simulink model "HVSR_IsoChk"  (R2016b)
settings: Solver=VariableStepAuto  StartTime=0.0  StopTime=10.0  RelTol=1e-3
undefined symbols (not defined in the file or in its folder): bin2dec, enmActv, enmBmsMode, enmCctErr, enmSWSta, HVSR_bIsoResShieldCal, HVSR_bSw1EnaByMnl_C, HVSR_bSw2EnaByMnl_C, HVSR_bSw3EnaByMnl_C, HVSR_bSwEnaByMnl_C, HVSR_bVldEnaByMnl_C, HVSR_cntIsoChkCnfDiag_C, HVSR_cntIsoChkCnfLv1Diag_C, HVSR_cntIsoChkDiag_CW, HVSR_cntPwrDown_C, HVSR_cofPosVoltfilter_C, HVSR_cofResGain_C, HVSR_deltInsRes_C, HVSR_InsResCtrlSw_C, HVSR_kSlopeVal_C, HVSR_numBgnTimeCnt_C, HVSR_numCycleTimeCnt_C, HVSR_numIsoCnst_C, HVSR_numSlopeCnfrm_C, HVSR_ResFirstCtrlSw_C, HVSR_resIsoFaultLvl1Thres_C, HVSR_resIsoFaultLvl2Thres_C, HVSR_ResR1_C, HVSR_ResR2_C, HVSR_ResR3_C, HVSR_resRstnUpLim_C, HVSR_rIsoCnfHysDiag_C, HVSR_rIsoCnfHysLv1Diag_C, HVSR_stBMSModeLvl_C, HVSR_tiChkFilteTime_C, HVSR_tiIsoChkCycl_T, HVSR_tiIsoChkDebounce_C, HVSR_tiIsoVldChkDebounce_C, HVSR_tiTaskTime_C, HVSR_tiVoltDiffThres_C, HVSR_uBattVoltRngHi_C, HVSR_uBattVoltRngLo_C, HVSR_uIsoKVoltThres_C, HVSR_uIsoPosVoltFilter_C, HVSR_uIsoVoltThres_C
libraries: simulink x78
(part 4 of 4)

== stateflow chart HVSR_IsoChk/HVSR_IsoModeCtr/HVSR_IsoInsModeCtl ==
  state Stt_init
    entry:
    HVSR_flgIsoChkStart = boolean(0);
    HVSR_stIsoStateObsr=uint8(0);
    HVSR_stIsoCctChkSta = enmCctDiagSta.DEFAULT;
    CctTotalTime = single(0);
  state Stt_CctChk
    entry:
    HVSR_flgIsoChkStart = boolean(0);
    HVSR_stIsoStateObsr=uint8(8);
    CctTotalTime = CctTotalTime+single(0.1);
    during:
    CctTotalTime = CctTotalTime+single(0.1);
    state Stt_CctChkInit
      entry:
      HVSR_stIsoCctChkSta = enmCctDiagSta.INIT;
      HVSR_numA1Val = single(0);
      HVSR_numA2Val = single(0);
      HVSR_numA3Val = single(0);
      HVSR_numA4Val = single(0);
      HVSR_numA5Val = single(0);
      HVSR_flgIsoCctChkOK = boolean(0);
      HVSR_stIsoCctChkErr = enmCctErr.DEFAULT;
      HVSR_bIsoChkSW1Sta = enmSWSta.SWOFF;
      HVSR_bIsoChkSW2Sta = enmSWSta.SWOFF;
      HVSR_bIsoChkSW3Sta = enmSWSta.SWOFF;
      CctCount = single(0);
    state Stt_CctChkA1
      entry:
      CctCount = single(0);
      HVSR_stIsoCctChkSta = enmCctDiagSta.A1CHK;
      HVSR_bIsoChkSW1Sta = enmSWSta.SWOFF;
      HVSR_bIsoChkSW2Sta = enmSWSta.SWOFF;
      HVSR_bIsoChkSW3Sta = enmSWSta.SWOFF;
      HVSR_numA1Val = BSPR_uIsoNegVolt/BSPR_uBattVolt;
      during:
      HVSR_numA1Val = BSPR_uIsoNegVolt/BSPR_uBattVolt;
      CctCount = CctCount + single(0.1);
    state Stt_CctChkA1Err
      entry:
      HVSR_bIsoChkSW1Sta = enmSWSta.SWOFF;
      HVSR_bIsoChkSW2Sta = enmSWSta.SWOFF;
      HVSR_bIsoChkSW3Sta = enmSWSta.SWOFF;
      HVSR_stIsoCctChkErr  = enmCctErr.CCTCLS;
      HVSR_stIsoCctChkSta = enmCctDiagSta.CCTERR;
      %S1或S2或S3常闭粘连
    state Stt_CctChkA2
      entry:
      CctCount = single(0);
      HVSR_stIsoCctChkSta = enmCctDiagSta.A2CHK;
      HVSR_bIsoChkSW1Sta = enmSWSta.SWON;
      HVSR_bIsoChkSW2Sta = enmSWSta.SWOFF;
      HVSR_bIsoChkSW3Sta = enmSWSta.SWOFF;
      HVSR_numA2Val = BSPR_uIsoNegVolt/BSPR_uBattVolt;
      during:
      HVSR_numA2Val = BSPR_uIsoNegVolt/BSPR_uBattVolt;
      CctCount = CctCount + single(0.1);
    state Stt_CctChkA2Err
      entry:
      HVSR_bIsoChkSW1Sta = enmSWSta.SWOFF;
      HVSR_bIsoChkSW2Sta = enmSWSta.SWOFF;
      HVSR_bIsoChkSW3Sta = enmSWSta.SWOFF;
      HVSR_stIsoCctChkErr = enmCctErr.S1ERR;
      HVSR_stIsoCctChkSta = enmCctDiagSta.CCTERR;
      %S1开关回路异常
    state Stt_CctChkA3
      entry:
      CctCount = single(0);
      HVSR_stIsoCctChkSta = enmCctDiagSta.A3CHK;
      HVSR_bIsoChkSW1Sta = enmSWSta.SWOFF;
      HVSR_bIsoChkSW2Sta = enmSWSta.SWON;
      HVSR_bIsoChkSW3Sta = enmSWSta.SWOFF;
      HVSR_numA3Val = BSPR_uIsoNegVolt/BSPR_uBattVolt;
      during:
      HVSR_numA3Val = BSPR_uIsoNegVolt/BSPR_uBattVolt;
      CctCount = CctCount + single(0.1);
    state Stt_CctChkA3Err
      entry:
      HVSR_bIsoChkSW1Sta = enmSWSta.SWOFF;
      HVSR_bIsoChkSW2Sta = enmSWSta.SWOFF;
      HVSR_bIsoChkSW3Sta = enmSWSta.SWOFF;
      HVSR_stIsoCctChkErr = enmCctErr.S2ERR;
      HVSR_stIsoCctChkSta = enmCctDiagSta.CCTERR;
      %S2开关回路异常
    state Stt_CctChkA4
      entry:
      CctCount = single(0);
      HVSR_stIsoCctChkSta = enmCctDiagSta.A4CHK;
      HVSR_bIsoChkSW1Sta = enmSWSta.SWOFF;
      HVSR_bIsoChkSW2Sta = enmSWSta.SWOFF;
      HVSR_bIsoChkSW3Sta = enmSWSta.SWON;
      HVSR_numA4Val = BSPR_uIsoNegVolt/BSPR_uBattVolt;
      during:
      HVSR_numA4Val = BSPR_uIsoNegVolt/BSPR_uBattVolt;
      CctCount = CctCount + single(0.1);
    state Stt_CctChkA4Err
      entry:
      CctCount = single(0);
      HVSR_stIsoCctChkSta = enmCctDiagSta.A5CHK;
      HVSR_bIsoChkSW1Sta = enmSWSta.SWON;
      HVSR_bIsoChkSW2Sta = enmSWSta.SWOFF;
      HVSR_bIsoChkSW3Sta = enmSWSta.SWON;
      HVSR_numA5Val = BSPR_uIsoNegVolt/BSPR_uBattVolt;
      during:
      HVSR_numA5Val = BSPR_uIsoNegVolt/BSPR_uBattVolt;
      CctCount = CctCount + single(0.1);
    state Stt_CctChkA5
      entry:
      HVSR_stIsoCctChkSta = enmCctDiagSta.A5CHK;
      HVSR_bIsoChkSW1Sta = enmSWSta.SWOFF;
      HVSR_bIsoChkSW2Sta = enmSWSta.SWOFF;
      HVSR_bIsoChkSW3Sta = enmSWSta.SWOFF;
      HVSR_flgIsoCctChkOK = boolean(1);
      HVSR_stIsoCctChkErr = enmCctErr.DEFAULT;
      %HVSR_stIsoCctChkErr = enmCctErr.S3ERR;
      HVSR_stIsoCctChkSta = enmCctDiagSta.CCTERR;
      %S3合不上或者Rp和Rn都非常大
    state Stt_CctChkA4OK
      entry:
      CctCount = single(0);
      HVSR_stIsoCctChkSta = enmCctDiagSta.A4CHK;
      HVSR_bIsoChkSW1Sta = enmSWSta.SWOFF;
      HVSR_bIsoChkSW2Sta = enmSWSta.SWOFF;
      HVSR_bIsoChkSW3Sta = enmSWSta.SWOFF;
    state Stt_CctChkA4OKRn
      entry:
      CctCount = single(0);
      HVSR_stIsoCctChkSta = enmCctDiagSta.CCTOK;
      HVSR_bIsoChkSW1Sta = enmSWSta.SWOFF;
      HVSR_bIsoChkSW2Sta = enmSWSta.SWOFF;
      HVSR_bIsoChkSW3Sta = enmSWSta.SWOFF;
      HVSR_flgIsoCctChkOK = boolean(1);
    state Stt_CctChkA4OKRp
      entry:
      CctCount = single(0);
      HVSR_stIsoCctChkSta = enmCctDiagSta.CCTOK;
      HVSR_bIsoChkSW1Sta = enmSWSta.SWOFF;
      HVSR_bIsoChkSW2Sta = enmSWSta.SWOFF;
      HVSR_bIsoChkSW3Sta = enmSWSta.SWOFF;
      HVSR_flgIsoCctChkOK = boolean(1);
    (default) -> Stt_CctChkInit
    Stt_CctChkInit -> Stt_CctChkA1
    Stt_CctChkA1 -> Stt_CctChkA1Err : [CctCount >HVSR_tiIsoCctChkWait_T]
    Stt_CctChkA1 -> Stt_CctChkA2 : [HVSR_numA1Val >=HVSR_numSwAllOpenMin_C &&...  HVSR_numA1Val <=HVSR_numSwAllOpenMax_C]
    Stt_CctChkA2 -> Stt_CctChkA2Err : [CctCount >HVSR_tiIsoCctChkWait_T]
    Stt_CctChkA2 -> Stt_CctChkA3 : [(HVSR_numA2Val >=HVSR_numSw1ClsdMin_C &&...  HVSR_numA2Val <=HVSR_numSw1ClsdMax_C)&&...  ((HVSR_numA2Val-HVSR_numA1Val) >= HVSR_numA1A2DiffMin_C &&... (HVSR_numA2Val-HVSR_numA1Val) <= HVSR_numA1A2DiffMax_C)]
    Stt_CctChkA3 -> Stt_CctChkA3Err : [CctCount >HVSR_tiIsoCctChkWait_T]
    Stt_CctChkA3 -> Stt_CctChkA4 : [(HVSR_numA3Val >=HVSR_numSw2ClsdMin_C &&...  HVSR_numA3Val <=HVSR_numSw2ClsdMax_C)&&... ((HVSR_numA1Val-HVSR_numA3Val) >= HVSR_numA1A3DiffMin_C &&... (HVSR_numA1Val-HVSR_numA3Val) <= HVSR_numA1A3DiffMax_C)]
    Stt_CctChkA4 -> Stt_CctChkA4Err : [CctCount >HVSR_tiIsoCctChkWait_T]
    Stt_CctChkA4 -> Stt_CctChkA4OK : [abs(HVSR_numA4Val-HVSR_numA1Val) >= HVSR_numA1A4Diff_C]
    Stt_CctChkA4Err -> Stt_CctChkA5 : [HVSR_numA5Val >=HVSR_numSw13ClsdMin_C &&...  HVSR_numA5Val <=HVSR_numSw13ClsdMax_C]
    Stt_CctChkA4OK -> (junction 191)
    (junction 191) -> Stt_CctChkA4OKRp
    Stt_CctChkA4OK -> Stt_CctChkA4OKRn : [(HVSR_numA4Val-HVSR_numA1Val) >= HVSR_numA1A4Diff_C]
  state Stt_fastchk
    entry:
    HVSR_flgIsoChkStart = boolean(0);
    HVSR_stIsoStateObsr=uint8(7);
  state Stt_standby
    entry:
    init_enable = enmActv.ACTIVE;
    begin_enable=enmActv.INACTIVE;
    control_enable=enmActv.INACTIVE;
    HVSR_flgIsoChkFault = boolean(0);
    HVSR_flgIsoChkStart = boolean(0);
    HVSR_stIsoStateObsr=uint8(1);
  state Stt_begin
    entry:
    init_enable = enmActv.INACTIVE;
    begin_enable=enmActv.ACTIVE;
    control_enable=enmActv.INACTIVE;
    HVSR_flgIsoChkStart = boolean(1);
    HVSR_flgInsResUpd = boolean(0);
    HVSR_stIsoStateObsr=uint8(2);
    counter = uint16(1);
    during:
    counter = counter + uint16(1);
  state Stt_work
    entry:
    init_enable = enmActv.INACTIVE;
    begin_enable=enmActv.INACTIVE;
    control_enable=enmActv.ACTIVE;
    HVSR_stIsoStateObsr=uint8(3);
  state Stt_fault
    entry:
    HVSR_flgIsoChkFault = boolean(1);
    HVSR_stIsoStateObsr=uint8(5);
  state 300 [group]
  state Stt_cycle
    entry:
    HVSR_flgInsResUpd = boolean(1);
    HVSR_flgIsoChkFault = boolean(0);
    HVSR_stIsoStateObsr=uint8(4);
    count = uint16(0);
    during:
    count =count + uint16(1);
  state Stt_end
    entry:
    init_enable = enmActv.ACTIVE;
    begin_enable=enmActv.INACTIVE;
    control_enable=enmActv.INACTIVE;
    HVSR_flgIsoChkStart = boolean(0);
    HVSR_stIsoStateObsr=uint8(6);
  (default) -> Stt_init
  Stt_init -> Stt_CctChk : [(BMCR_stBmsModeCtrl >= uint8(2))&&(BMCR_stBmsModeCtrl<=HVSR_ModLvl_C)]
  Stt_CctChk -> Stt_fastchk : [boolean(1) == HVSR_flgIsoCctChkOK||... CctTotalTime >= HVSR_tiIsoCctChkTotMax_T||... HVSR_bIsoCctChkEna_C]
  Stt_fastchk -> Stt_standby
  (junction 115) -> Stt_standby
  (junction 112) -> (junction 115)
  Stt_standby -> Stt_begin : [IsoResCalShieldCmd==boolean(0)]
  Stt_begin -> (junction 112) : [IsoResCalShieldCmd==1]
  (junction 109) -> (junction 112)
  (junction 86) -> Stt_begin
  (junction 50) -> Stt_begin
  Stt_fault -> (junction 86) : [BMCR_stBmsModeCtrl<=HVSR_ModLvl_C]
  (junction 48) -> (junction 50)
  Stt_begin -> (junction 47) : [(counter>HVSR_BgTi_C)&&(HVSR_flgFrstRsVlotVld==1)]
  (junction 47) -> Stt_work : {HVSR_cntPwrDown = uint16(0)}
  (junction 43) -> Stt_work : {HVSR_cntPwrDown = HVSR_cntPwrDown + 1}
  (junction 39) -> (junction 43)
  Stt_work -> Stt_fault : [(flgResVald == 0)&&(HVSR_cntPwrDown > HVSR_cntPwrDown_C)]
  Stt_work -> (junction 39) : [(flgResVald == 0)&&(HVSR_cntPwrDown <= HVSR_cntPwrDown_C)]
  Stt_work -> (junction 109) : [IsoResCalShieldCmd==1]
  (junction 105) -> (junction 109)
  Stt_fault -> (junction 89) : [BMCR_stBmsModeCtrl >HVSR_ModLvl_C]
  Stt_work -> Stt_cycle : [flgResVald == boolean(1)]
  Stt_cycle -> (junction 48) : [(BMCR_stBmsModeCtrl <= HVSR_ModLvl_C)&&(count > HVSR_CycleTi_C)]
  Stt_cycle -> (junction 105) : [IsoResCalShieldCmd==1]
  Stt_cycle -> Stt_end : [BMCR_stBmsModeCtrl >HVSR_ModLvl_C]
  (junction 89) -> Stt_end
  data: HVSR_numA1Val output single; HVSR_numA2Val output single; HVSR_numA3Val output single; HVSR_numA4Val output single; HVSR_numA5Val output single; HVSR_flgIsoCctChkOK output boolean; HVSR_stIsoCctChkErr output Enum: enmCctErr; HVSR_stIsoCctChkSta output Enum: enmCctDiagSta; HVSR_flgIsoChkStart output boolean; HVSR_flgIsoChkFault output boolean; HVSR_flgInsResUpd output boolean; HVSR_stIsoStateObsr output uint8; control_enable output Enum: enmActv; HVSR_cntPwrDown local uint16; flgResVald input boolean; init_enable output Enum: enmActv; begin_enable output Enum: enmActv; counter local uint16; count local uint16; HVSR_BgTi_C input uint16; HVSR_CycleTi_C input uint16; HVSR_ModLvl_C input uint8; BMCR_stBmsModeCtrl input uint8; HVSR_flgFrstRsVlotVld input boolean; IsoResCalShieldCmd input boolean; HVSR_cntPwrDown_C input uint16; HVSR_bIsoChkSW1Sta output Enum: enmSWSta; HVSR_bIsoChkSW2Sta output Enum: enmSWSta; HVSR_bIsoChkSW3Sta output Enum: enmSWSta; BSPR_uIsoNegVolt input single; BSPR_uBattVolt input single; HVSR_numSwAllOpenMin_C parameter; HVSR_numSwAllOpenMax_C parameter; HVSR_numSw1ClsdMin_C parameter; HVSR_numSw1ClsdMax_C parameter; HVSR_numA1A2DiffMin_C parameter; HVSR_numA1A2DiffMax_C parameter; HVSR_numSw2ClsdMin_C parameter; HVSR_numSw2ClsdMax_C parameter; HVSR_numA1A3DiffMin_C parameter; HVSR_numA1A3DiffMax_C parameter; HVSR_numA1A4Diff_C parameter; HVSR_numSw13ClsdMin_C parameter; HVSR_numSw13ClsdMax_C parameter; CctCount local single; HVSR_tiIsoCctChkWait_T parameter single; CctTotalTime local single; HVSR_tiIsoCctChkTotMax_T parameter single; HVSR_bIsoCctChkEna_C parameter boolean

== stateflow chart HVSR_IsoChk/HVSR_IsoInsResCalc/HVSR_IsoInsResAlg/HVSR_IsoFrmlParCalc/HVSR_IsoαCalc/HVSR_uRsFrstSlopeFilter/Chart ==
  state Fast_mode_init
    entry:
    ISOFilterSta = uint8(1);
    Slope_RS = single(100);
    cnt = uint8(0);
    tc = HVSR_tiIsoChkCycl_T;
    HVSR_bSlopeVld =  0;
  state Fast_mode_filter
    entry:
    ISOFilterSta = uint8(2);
    Slope_RS = single(100);
    cnt = uint8(0);
    HVSR_bSlopeVld =  0;
    exit:
    cnt = uint8(0);
    (default) -> (junction 237) : { Temp1 = single(0); KIRS_filter_slope = uint8(0); }
    Fast_mode_filter -> (junction 237) : {Temp1 = V1;}
    (junction 237) -> (junction 228) : [abs(Slope_RS) < HVSR_kSlopeVal]
    (junction 237) -> (junction 243) : { V1 = single(HVSR_uIsoRsVolt); KIRS_filter_slope = uint8(0); 	 }
    (junction 228) -> (junction 235) : {KIRS_filter_slope = KIRS_filter_slope + 1;}
    (junction 243) -> (junction 235) : [cnt > 0]
    (junction 235) -> (junction 236) : [KIRS_filter_slope > HVSR_numSlopeCnfrm]
    (junction 243) -> (junction 241) : {cnt = cnt + 1;}
    (junction 235) -> (junction 239) : { V1 = single(HVSR_uIsoRsVolt); Delta_RS = V1 - Temp1; Slope_RS = Delta_RS/tc; cnt = cnt + 1; }
    (junction 236) -> (junction 229) : {HVSR_bSlopeVld = 1;}
    (junction 239) -> (junction 241)
    (junction 229) -> (junction 239)
  state Fast_mode_end
    entry:
    ISOFilterSta = uint8(3);
    exit:
  (default) -> Fast_mode_init
  Fast_mode_init -> Fast_mode_filter
  Fast_mode_filter -> Fast_mode_end : [HVSR_bSlopeVld == 1]
  data: HVSR_bSlopeVld output boolean; HVSR_uIsoRsVolt input single; Temp1 local single; Slope_RS local single; Temp2 local single; V1 local single; HVSR_kSlopeVal input single; KIRS_filter_slope local uint8; cnt local uint8; V2 local single; Slope_VB local single; HVSR_tiIsoChkCycl_T input single; ISOFilterSta output uint8; tc local single; HVSR_numSlopeCnfrm input uint8; Delta_RS local single

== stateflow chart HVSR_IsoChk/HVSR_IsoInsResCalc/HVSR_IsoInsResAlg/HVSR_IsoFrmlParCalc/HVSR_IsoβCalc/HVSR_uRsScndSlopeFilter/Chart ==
  state Fast_mode_init
    entry:
    ISOFilterSta = uint8(1);
    Slope_RS = single(100);
    cnt = uint8(0);
    tc = HVSR_tiIsoChkCycl_T;
    HVSR_bSlopeVld =  0;
  state Fast_mode_filter
    entry:
    ISOFilterSta = uint8(2);
    Slope_RS = single(100);
    cnt = uint8(0);
    HVSR_bSlopeVld =  0;
    exit:
    cnt = uint8(0);
    (default) -> (junction 237) : { Temp1 = single(0); KIRS_filter_slope = uint8(0); }
    Fast_mode_filter -> (junction 237) : {Temp1 = V1;}
    (junction 237) -> (junction 228) : [abs(Slope_RS) < HVSR_kSlopeVal]
    (junction 237) -> (junction 243) : { V1 = single(HVSR_uIsoRsVolt); KIRS_filter_slope = uint8(0); 	 }
    (junction 228) -> (junction 235) : {KIRS_filter_slope = KIRS_filter_slope + 1;}
    (junction 243) -> (junction 235) : [cnt > 0]
    (junction 235) -> (junction 236) : [KIRS_filter_slope > HVSR_numSlopeCnfrm]
    (junction 243) -> (junction 241) : {cnt = cnt + 1;}
    (junction 235) -> (junction 239) : { V1 = single(HVSR_uIsoRsVolt); Delta_RS = V1 - Temp1; Slope_RS = Delta_RS/tc; cnt = cnt + 1; }
    (junction 236) -> (junction 229) : {HVSR_bSlopeVld = 1;}
    (junction 239) -> (junction 241)
    (junction 229) -> (junction 239)
  state Fast_mode_end
    entry:
    ISOFilterSta = uint8(3);
    exit:
  (default) -> Fast_mode_init
  Fast_mode_init -> Fast_mode_filter
  Fast_mode_filter -> Fast_mode_end : [HVSR_bSlopeVld == 1]
  data: HVSR_bSlopeVld output boolean; HVSR_uIsoRsVolt input single; Temp1 local single; Slope_RS local single; Temp2 local single; V1 local single; HVSR_kSlopeVal input single; KIRS_filter_slope local uint8; cnt local uint8; V2 local single; Slope_VB local single; HVSR_tiIsoChkCycl_T input single; ISOFilterSta output uint8; tc local single; HVSR_numSlopeCnfrm input uint8; Delta_RS local single
